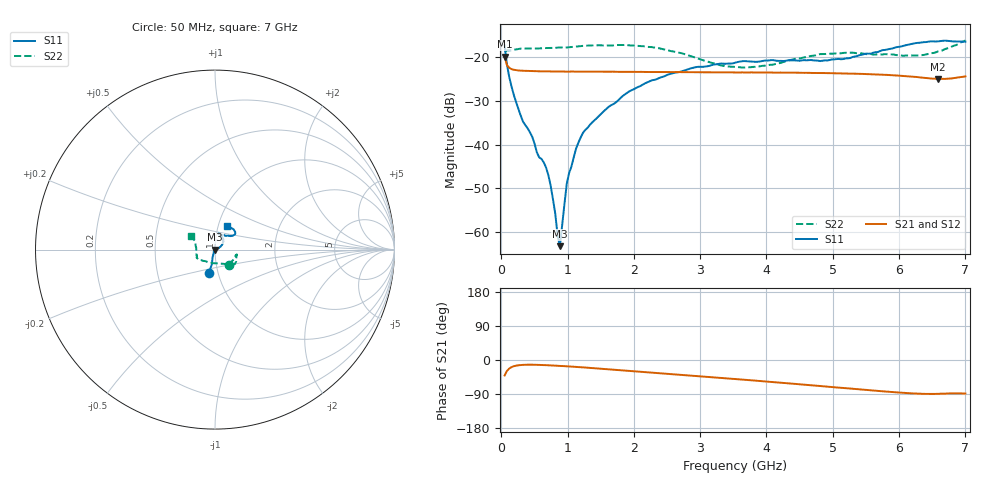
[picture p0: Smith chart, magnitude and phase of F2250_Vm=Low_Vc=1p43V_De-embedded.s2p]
! Integrated Device Technology
! Corporate Headquarters
! 6024 Silver Creek Valley Road
! San Jose, CA 95138  USA
! Phone:  1-408-284-8200
! Toll Free:  1-800-223-1366
! Webpage:  http://www.idt.com/
! Timing and RF Division
! 515 Groton Road, Suite 102
! Westford, MA 01886-6024
! Device:  F2250
! Description: Voltage Variable RF Attenuator
! Frequency:  50.0 -  6000.00 MHz
! Package:  3x3 mm Thin QFN Plastic Package: 16 pin
! Ports:  2 RF, 3 DC
!  Pin  1  = GND
!  Pin  2  = NC
!  Pin  3  = RF1  = Port 1
!  Pin  4  = NC
!  Pin  5  = GND
!  Pin  6  = GND
!  Pin  7  = GND
!  Pin  8  = GND
!  Pin  9  = NC
!  Pin 10  = RF2  = Port 2
!  Pin 11  = NC
!  Pin 12  = GND
!  Pin 13  = GND
!  Pin 14  = VCNTRL
!  Pin 15  = VDD
!  Pin 16  = VMODE
! Vcntrl:  1.430 Volts
! Vmode:  +0.000 Volts
! Vdd:  +3.30  Volts
! Current:  1.191 mA
! Data:  The device was measured on a the F2250 evaluation board which has
!  individual transmission lines to the RF pins.  Data was collected
!  using a calibrated network analyzer.  The evaluation board was
!  de-embedded using a TRL calibration technique.
!  The reference plane is the edge of the package pin.
! Misc:  SN 10
!  Action Tracker AT0258
! Date Measured:  2014-11-26
! Date:  2015-10-15  MJV
! Note:
!  Integrated Device Technology supplies this data as a sample of measured
!  data at the package pin for this product.  Your particular data for this
!  product may vary.
!  Data was taken at 25 degrees C.
!  Integrated Device Technology reserves the right to change this data at anytime.
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# GHz S dB R 50
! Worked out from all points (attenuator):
!   201 points, 50 MHz to 7 GHz, reference 50 ohm
!   highest |S21| = -19.93 dB at 50 MHz (marker M1); lowest = -25.0 dB at 6.583 GHz (marker M2)
!   lowest |S11| = -63.2 dB at 884 MHz (marker M3), VSWR 1.00, Z = 50.1 - j0.0468 ohm
!   |S11| at or under -10 dB: start of sweep to end of sweep
!   |S22| runs from -22.4 to -16.2 dB; largest |S21 - S12| = 0.00028
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0.05  -17.34 -105.0  -19.93 -40.9  -19.92 -40.8  -18.89 -48.2
0.1195  -24.55 -104.5  -22.47 -22.5  -22.48 -22.5  -18.49 -18.3
0.22375  -30.32 -109.0  -23.02 -14.9  -23.02 -14.9  -18.28 -13.6
0.328  -34.77 -113.9  -23.15 -12.8  -23.15 -12.8  -18.08 -12.6
0.467  -38.22 -122.2  -23.22 -12.4  -23.22 -12.4  -18.10 -13.6
0.5365  -41.76 -122.8  -23.27 -12.7  -23.27 -12.7  -18.08 -15.0
0.64075  -44.07 -121.3  -23.29 -13.4  -23.29 -13.4  -17.99 -16.9
0.71025  -46.97 -120.5  -23.30 -13.9  -23.28 -13.9  -17.96 -18.5
0.77975  -52.50 -136.6  -23.31 -14.5  -23.31 -14.5  -17.95 -19.9
0.8145  -55.78 -142.7  -23.32 -14.9  -23.31 -14.9  -17.92 -20.8
0.84925  -60.73 -120.5  -23.32 -15.2  -23.31 -15.2  -17.87 -21.6
0.884  -63.16 -42.3  -23.32 -15.6  -23.32 -15.5  -17.86 -22.3
0.98825  -48.86 -18.4  -23.34 -16.6  -23.34 -16.6  -17.84 -24.1
1.12725  -40.93 7.3  -23.35 -18.2  -23.32 -18.2  -17.64 -26.3
1.2315  -37.31 12.8  -23.33 -19.4  -23.33 -19.4  -17.47 -28.3
1.857  -28.62 29.3  -23.40 -27.5  -23.41 -27.5  -17.28 -35.6
2.37825  -24.83 39.9  -23.44 -34.4  -23.43 -34.4  -18.02 -41.7
3.525  -21.32 69.1  -23.53 -50.2  -23.54 -50.2  -22.26 -89.2
4.7065  -20.79 70.6  -23.66 -67.1  -23.64 -67.2  -19.72 -146.8
5.85325  -18.19 38.6  -24.12 -83.9  -24.12 -84.0  -19.45 -165.6
6.583  -16.45 44.5  -25.03 -89.3  -25.02 -89.4  -18.75 162.6
7  -16.51 62.7  -24.44 -88.4  -24.44 -88.5  -16.24 150.4
